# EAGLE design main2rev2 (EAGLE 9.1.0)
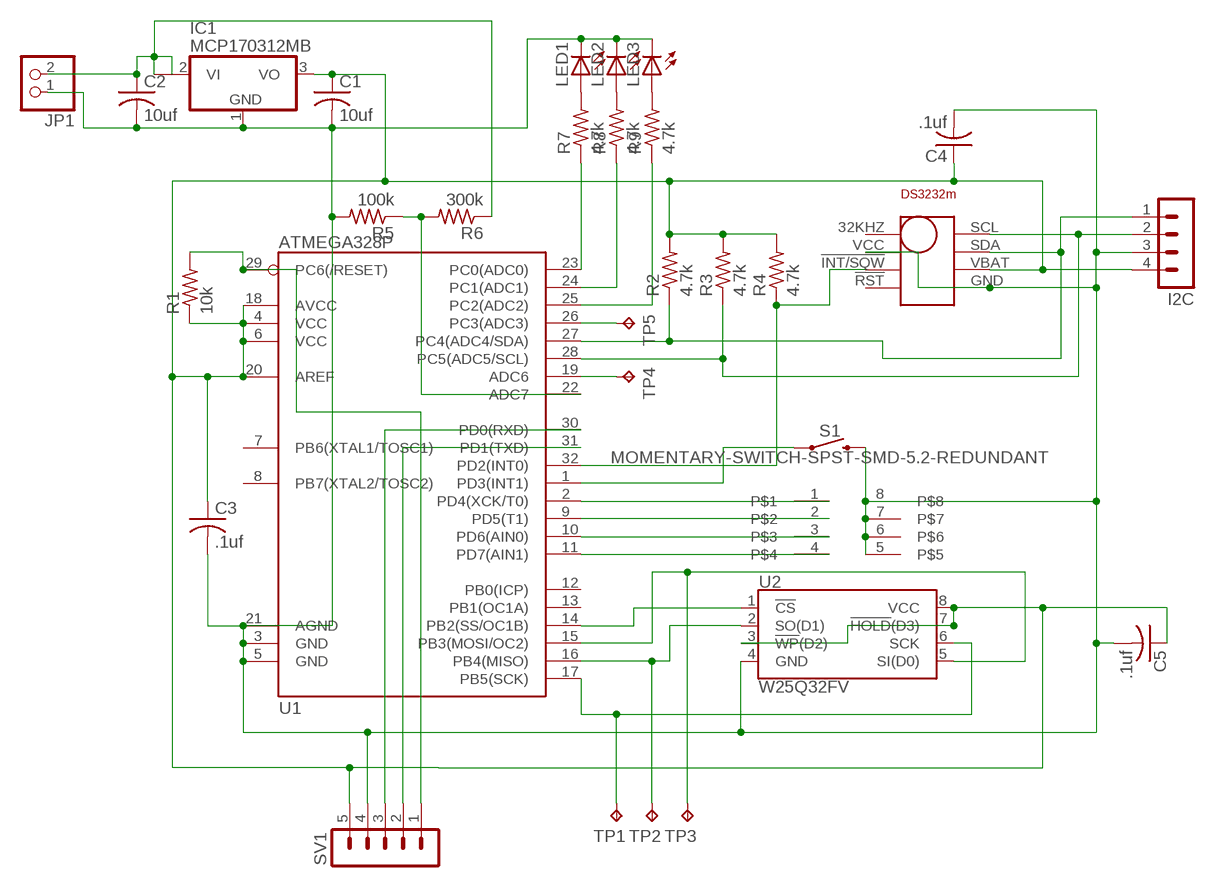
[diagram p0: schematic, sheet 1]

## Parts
C1  10uf  C-USC0805K  [C0805K]
C2  10uf  C-USC0805K  [C0805K]
C3  .1uf  C-USC0805K  [C0805K]
C4  .1uf  C-USC0805K  [C0805K]
C5  .1uf  C-USC0805K  [C0805K]
I2C  MA04-1  [MA04-1]
IC1  MCP170312MB  [SOT89]
JP1  PINHD-1X2  [1X02]
LED1  LEDSML0805  [SML0805]
LED2  LEDSML0805  [SML0805]
LED3  LEDSML0805  [SML0805]
R1  10k  R-US_R0805  [R0805]
R2  4.7k  R-US_R0805  [R0805]
R3  4.7k  R-US_R0805  [R0805]
R4  4.7k  R-US_R0805  [R0805]
R5  100k  R-US_R0805  [R0805]
R6  300k  R-US_R0805  [R0805]
R7  4.7k  R-US_R0805  [R0805]
R8  4.7k  R-US_R0805  [R0805]
R9  4.7k  R-US_R0805  [R0805]
S1  MOMENTARY-SWITCH-SPST-SMD-5.2-REDUNDANT  [TACTILE_SWITCH_SMD_5.2MM]
SV1  MA05-1  [MA05-1]
TP1  TPB1,27  [B1,27]
TP2  TPB1,27  [B1,27]
TP3  TPB1,27  [B1,27]
TP4  TPB1,27  [B1,27]
TP5  TPB1,27  [B1,27]
U1  ATMEGA328P  ATMEGA328_SMT  [TQFP32-08]
U2  W25Q32FV  W25Q32FVSS  [SOIC-8]
U$1  DS3232M  [SOIC8]
U$2  SO8-208  [SO08-208]

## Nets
N$1: S1.1 S1.2 U1.1(PD3(INT1))
N$2: TP1.TP U1.17(PB5(SCK)) U2.6(SCK)
N$3: R4.1 U1.32(PD2(INT0)) U$1.!INT/!!SQW
N$4: R1.2 SV1.1 U1.29(PC6(/RESET))
N$5: TP3.TP U1.15(PB3(MOSI/OC2)) U2.5(SI(D0))
N$6: TP2.TP U1.16(PB4(MISO)) U2.2(SO(D1))
N$7: U1.14(PB2(SS/OC1B)) U2.1(!CS!)
N$8: I2C.1 R2.1 U1.27(PC4(ADC4/SDA)) U$1.SDA
N$9: I2C.2 R3.1 U1.28(PC5(ADC5/SCL)) U$1.SCL
N$10: SV1.3 U1.30(PD0(RXD))
N$11: U1.11(PD7(AIN1)) U$2.4
N$12: U1.10(PD6(AIN0)) U$2.3
N$13: U1.9(PD5(T1)) U$2.2
N$14: U1.2(PD4(XCK/T0)) U$2.1
N$15: C1.2 C2.2 C3.2 C4.2 C5.2 I2C.3 IC1.1(GND) JP1.1 LED1.C LED2.C LED3.C R5.2 S1.3 S1.4 SV1.4 U1.3(GND) U1.5(GND) U1.21(AGND) U2.4(GND) U$1.GND U$1.VCC U$2.5 U$2.6 U$2.7 U$2.8
N$16: SV1.2 U1.31(PD1(TXD))
N$18: R5.1 R6.2 U1.22(ADC7)
N$19: LED1.A R7.2
N$20: LED2.A R8.2
N$21: LED3.A R9.2
N$22: R7.1 U1.23(PC0(ADC0))
N$23: R8.1 U1.24(PC1(ADC1))
N$24: R9.1 U1.25(PC2(ADC2))
N$25: C2.1 IC1.2(VI) IC1.2@1(VI1) JP1.2 R6.1
N$26: TP4.TP U1.19(ADC6)
N$27: C1.1 C3.1 C4.1 C5.1 I2C.4 IC1.3(VO) R1.1 R2.2 R3.2 R4.2 SV1.5 U1.4(VCC) U1.6(VCC) U1.18(AVCC) U1.20(AREF) U2.3(!WP!(D2)) U2.7(!HOLD!(D3)) U2.8(VCC) U$1.VBAT
N$28: TP5.TP U1.26(PC3(ADC3))
Unconnected: U1.7(PB6(XTAL1/TOSC1)) U1.8(PB7(XTAL2/TOSC2)) U1.12(PB0(ICP)) U1.13(PB1(OC1A)) U$1.32KHZ U$1.!RST

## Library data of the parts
C1-C5 = resistor:C-US: CAPACITOR, American symbol
I2C = con-lstb:MA04-1: PIN HEADER; OC_FARNELL: unknown; OC_NEWARK: unknown
IC1 = linear:MCP1703*: 250 mA, 16V, Low Quiescent Current LDO Regulator Source: http://ww1.microchip.com/downloads/en/DeviceDoc/22049b.pdf
JP1 = pinhead:PINHD-1X2: PIN HEADER
LED1-LED3 = led:LED: LED
R1-R9 = resistor:R-US_: RESISTOR, American symbol
S1 = SparkFun-Switches:MOMENTARY-SWITCH-SPST: Momentary Switch (Pushbutton) - SPST; PROD_ID: SWCH-08247; SF_SKU: COM-08720
SV1 = con-lstb:MA05-1: PIN HEADER; OC_FARNELL: unknown; OC_NEWARK: unknown
TP1-TP5 = testpad:TP: Test pad
U1 = SparkFun-DigitalIC:ATMEGA328_SMT: 32-Pin Atmega328 part Commonly used on Arduino compatible boards Available in QFP and QFN packages TQFP is IC-09069 QFN is non-stock; PROD_ID: IC-09069
U2 = SparkFun-IC-Memory:W25Q32FV: W25Q32FV 32Mb (4MB) Serial Flash Memory The W25Q32FV support the standard Serial Peripheral Interface (SPI), Dual/Quad I/O SPI as well as 2-clocks instruction cycle Quad Peripheral Interface (QPI). 104MHz, SPI, 8-SOIC-EIAJ Datasheet SparkFun Products SparkFun Blynk Board - ESP8266 (WRL-13794); PROD_ID: IC-13229
U$1 = DS3232M:DS3232M
U$2 = IC-packages_BIG-pack V1.0:SO8-208

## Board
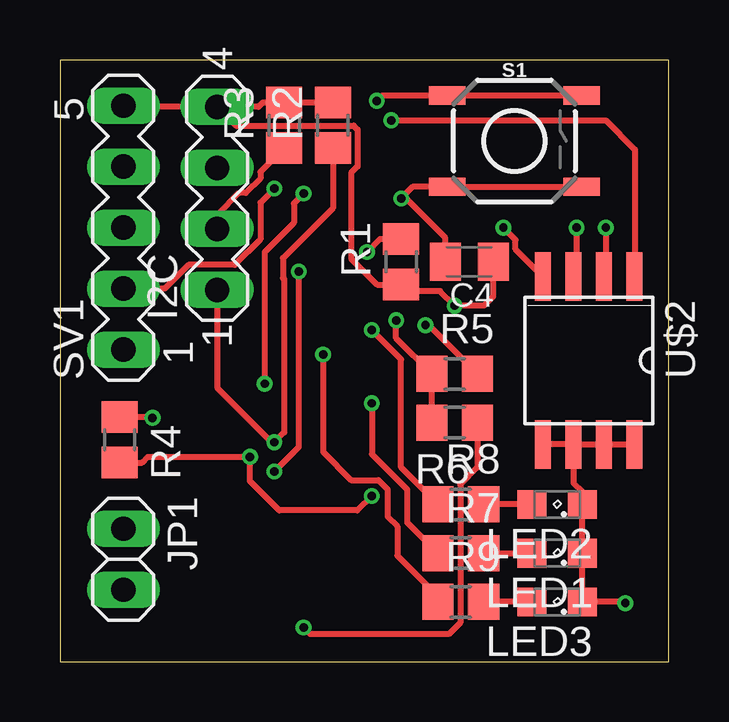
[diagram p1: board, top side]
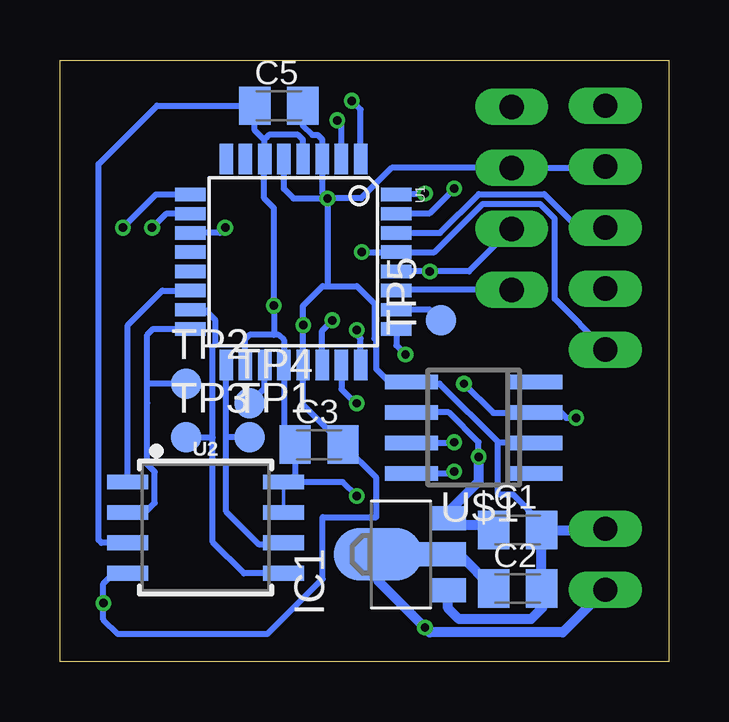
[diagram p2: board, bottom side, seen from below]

Size 25.38 x 25.07 mm. Coordinates in mm from the lower left corner, seen from the top.
Outline: 0,0 25.38,0 25.38,25.07 0,25.07 0,0
Copper layers (1*16): Top 0.035mm / dielectric 1.5mm / Bottom 0.035mm
Design rules "dirt_cheap_dirty_boards.v1.1": minimum track width 6mil, minimum drill 12mil, track to track 6mil, track to pad 6mil, pad to pad 6mil, via to via 6mil, smd to smd 0mil, copper to edge 10mil, drill to drill 10mil, minimum pad ring 10mil, minimum via ring 6mil, stop-mask expansion 2mil, vias tented up to drill 25mil, thermal gap 10mil

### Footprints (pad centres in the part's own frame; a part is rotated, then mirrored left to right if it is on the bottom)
C0805K = smd 1.3 x 1.6: 1 -1,0; 2 1,0
MA04-1 = drill 1.016 long: 1 -3.81,0; 2 -1.27,0; 3 1.27,0; 4 3.81,0
SOT89 = smd 1 x 1.5: 1 -1.499,-1.981; 3 1.499,-1.981 | smd 1 x 2: 2 0,-1.727 | smd 2.2 x 3.7: 2@1 0,0.94
1X02 = drill 1.016 long: 1 -1.27,0; 2 1.27,0
SML0805 = smd 1.2 x 1.2: A 1.05,0; C -1.05,0
R0805 = smd 1.3 x 1.5: 1 -0.95,0; 2 0.95,0
TACTILE_SWITCH_SMD_5.2MM = smd 1.524 x 0.762: 1 -2.794,1.905; 2 2.794,1.905; 3 -2.794,-1.905; 4 2.794,-1.905
MA05-1 = drill 1.016 long: 1 -5.08,0; 2 -2.54,0; 3 0,0; 4 2.54,0; 5 5.08,0
B1,27 = smd 1.27 x 1.27: TP 0,0
TQFP32-08 = smd 1.27 x 0.559: 1 -4.293,2.8; 2 -4.293,2; 3 -4.293,1.2; 4 -4.293,0.4; 5 -4.293,-0.4; 6 -4.293,-1.2; 7 -4.293,-2; 8 -4.293,-2.8; 17 4.293,-2.8; 18 4.293,-2; 19 4.293,-1.2; 20 4.293,-0.4; 21 4.293,0.4; 22 4.293,1.2; 23 4.293,2; 24 4.293,2.8 | smd 0.559 x 1.27: 9 -2.8,-4.293; 10 -2,-4.293; 11 -1.2,-4.293; 12 -0.4,-4.293; 13 0.4,-4.293; 14 1.2,-4.293; 15 2,-4.293; 16 2.8,-4.293; 25 2.8,4.293; 26 2,4.293; 27 1.2,4.293; 28 0.4,4.293; 29 -0.4,4.293; 30 -1.2,4.293; 31 -2,4.293; 32 -2.8,4.293
SOIC-8 = smd 0.61 x 1.702: 1 -1.905,-3.251; 2 -0.635,-3.251; 3 0.635,-3.251; 4 1.905,-3.251; 5 1.905,3.251; 6 0.635,3.251; 7 -0.635,3.251; 8 -1.905,3.251
SOIC8 = smd 0.6 x 2.2: 32KHZ -1.905,-2.6; !INT/!!SQW 0.635,-2.6; !RST 1.905,-2.6; GND 1.905,2.6; SCL -1.905,2.6; SDA -0.635,2.6; VBAT 0.635,2.6; VCC -0.635,-2.6
SO08-208 = smd 0.66 x 2.032: 1 -1.905,-3.498; 2 -0.635,-3.498; 3 0.635,-3.498; 4 1.905,-3.498; 5 1.905,3.498; 6 0.635,3.498; 7 -0.635,3.498; 8 -1.905,3.498

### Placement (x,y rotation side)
C1  6.3,5.49 0 bottom
C2  6.3,3.05 0 bottom
C3  14.58,9.04 0 bottom
C4  17.07,16.66 180 top
C5  16.26,23.16 0 bottom
I2C  6.55,19.3 90 top
IC1  11.18,4.47 90 bottom
JP1  2.64,4.27 270 top
LED1  20.73,4.52 180 top
LED2  20.73,6.55 180 top
LED3  20.73,2.49 180 top
R1  14.22,16.66 90 top
R2  11.38,22.35 90 top
R3  9.35,22.35 90 top
R4  2.49,9.25 270 top
R5  16.46,11.99 0 top
R6  16.46,9.96 180 top
R7  16.71,4.52 0 top
R8  16.71,6.55 0 top
R9  16.71,2.49 0 top
S1  18.95,21.69 0 top
SV1  2.64,18.08 90 top
TP1  17.48,9.35 0 bottom
TP2  20.12,11.58 0 bottom
TP3  20.12,9.35 0 bottom
TP4  17.48,10.77 0 bottom
TP5  9.5,14.22 90 bottom
U1  15.65,16.66 270 bottom
U2  19.3,5.59 270 bottom
U$1  8.13,9.75 90 bottom
U$2  22.05,12.55 180 top

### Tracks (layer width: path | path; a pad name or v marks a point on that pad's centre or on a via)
N$1  (via drill 0.35)
  Top 0.254: v13.21,23.37 13.44,23.6 S1.1 S1.2
  Bottom 0.254: U1.1 12.85,23.01 v13.21,23.37
N$2
  Bottom 0.254: U2.6 16.13,4.88 17.07,4.88 18.45,6.25 18.45,9.35 | 18.45,9.35 U1.17 | TP1.TP 18.45,9.35
N$3  (via drill 0.35)
  Top 0.254: v10.16,19.51 9.75,19.1 9.75,18.29 8.53,17.07 v8.53,11.58 | R4.1 3.83,10.2 v3.86,10.16
  Bottom 0.254: U1.32 11.31,19.51 v10.16,19.51 | v8.53,11.58 7.32,10.36 5.55,10.36 U$1.!INT/!!SQW 4.5,10.39 4.27,10.16 v3.86,10.16
N$4  (via drill 0.35)
  Top 0.254: v12.8,17.07 13.35,17.61 R1.2
  Bottom 0.254: v12.8,17.07 U1.29 9.76,17.06 7.75,19.07 5.36,19.07 4.75,18.46 4.75,15.11 SV1.1
N$5
  Bottom 0.254: U2.5 17.7,3.68 19,4.98 19,9.35 | 19,9.35 19,13.12 18.9,13.23 18.9,14.22 19.34,14.66 U1.15 | TP3.TP 19,9.35
N$6
  Bottom 0.254: U2.2 21.82,6.22 21.43,6.62 21.43,7.91 21.74,8.23 21.74,10.77 21.74,11.58 | 21.74,11.58 21.74,13.61 21.49,13.86 U1.16 | TP2.TP 21.74,11.58
N$7
  Bottom 0.254: U2.1 22.55,14.02 21.11,15.46 U1.14
N$8  (via drill 0.35)
  Top 0.254: I2C.1 6.55,11.41 8.82,9.14 v8.94,9.14 9.35,9.55 9.35,15.94 9.3,15.98 9.3,16.82 11.38,18.9 R2.1
  Bottom 0.254: I2C.1 11.32,15.49 U1.27 | U$1.SDA 8.91,9.12 v8.94,9.14
N$9  (via drill 0.35)
  Top 0.254: I2C.2 6.55,18.61 7.48,19.53 7.75,19.53 8.36,20.14 8.36,20.41 R3.1 | v9.96,16.26 9.96,8.94 v8.94,7.92
  Bottom 0.254: I2C.2 8.32,16.26 v9.95,16.26 v9.96,16.26 U1.28 | v8.94,7.92 9.02,7.85 U$1.SCL
N$10
  Bottom 0.254: SV1.3 2.86,17.86 3.57,17.86 5.19,19.48 7.92,19.48 9.53,17.86 U1.30
N$11  (via drill 0.35)
  Top 0.254: U$2.4 19,17.19 19,17.58 v18.49,18.09 | v18.49,18.09
  Bottom 0.254: v18.49,18.09 18.71,17.86 U1.11
N$12  (via drill 0.35)
  Top 0.254: v21.54,18.09 21.54,16.17 U$2.3
  Bottom 0.254: U1.10 20.96,18.66 v21.54,18.09
N$13  (via drill 0.35)
  Top 0.254: v22.76,18.09 22.76,16.12 U$2.2
  Bottom 0.254: U1.9 21.38,19.46 v22.76,18.09
N$14  (via drill 0.35)
  Top 0.254: v13.82,22.55 22.76,22.55 23.98,21.34 23.98,16.07 U$2.1
  Bottom 0.254: U1.2 13.65,22.38 v13.82,22.55
N$15  (via drill 0.35)
  Top 0.254: C4.2 16.07,17.66 14.43,19.3 v14.22,19.3 14.71,19.79 S1.3 S1.4 | R5.2 15.38,14.02 v15.24,14.02 | U$2.6 21.41,7.44 21.78,7.08 LED2.C LED1.C LED3.C 23.52,2.49 v23.57,2.44 | U$2.6 U$2.5 | U$2.6 U$2.7 U$2.8
  Bottom 0.254: U$1.VCC 7.09,9.12 | 7.09,9.12 7.11,9.09 7.11,6.97 6.5,6.97 5.3,5.77 C1.2 | U1.5 16.05,19.7 15.65,19.3 v14.22,19.3 | C5.2 15.26,22.33 14.87,21.95 14.63,21.95 14.45,21.76 U1.3 14.43,20.94 14.43,19.51 v14.22,19.3 | SV1.4 2.69,20.57 I2C.3 11.55,20.57 12.82,19.3 v14.22,19.3 | 14.43,3.45 | 7.09,9.12 9.55,11.58 9.96,11.58 10.03,11.66 U$1.GND 11.66,11.66 12.19,12.19 12.19,13.39 12.27,13.47 12.27,14.91 13.01,15.65 14.22,15.65 | 14.22,15.65 14.43,15.65 15.25,14.83 | 15.25,14.83 | 15.25,14.83 15.24,14.82 v15.24,14.02 v15.25,14.01 U1.21 15.24,10.7 C3.2 12.19,7.66 12.19,6.02 14.43,6.02 14.43,3.45 | 14.43,3.45 | 14.43,3.45 | 14.43,3.45 16.74,1.14 22.96,1.14 23.57,1.75 v23.57,2.44 23.57,3.25 23.14,3.68 U2.4 | v14.22,19.3 14.22,15.65
  Bottom 0.406: IC1.1 9.2,2.23 8.74,1.78 5.74,1.78 5.28,2.23 5.3,2.25 C2.2 C1.2 2.69,5.49 JP1.1
N$16  (via drill 0.35)
  Top 0.254: v8.94,19.71 8.36,19.13 8.36,17.6 7.29,16.54 5.36,16.54 4.37,15.54 SV1.2
  Bottom 0.254: U1.31 11.32,18.69 9.96,18.69 v8.94,19.71
N$18  (via drill 0.35)
  Top 0.254: v14.02,14.22 14.02,13.48 R5.1 R6.2
  Bottom 0.254: U1.22 14.45,13.8 v14.02,14.22
N$19
  Top 0.254: R7.2 LED1.A
N$20
  Top 0.254: LED2.A R8.2
N$21
  Top 0.254: LED3.A R9.2
N$22  (via drill 0.35)
  Top 0.254: v13.01,10.77 13.01,8.65 14.47,7.18 14.47,5.81 R7.1
  Bottom 0.254: v13.01,10.77 13.06,10.77 13.65,11.35 U1.23
N$23  (via drill 0.35)
  Top 0.254: R8.1 14.22,8.09 14.22,12.6 v13.01,13.82
  Bottom 0.254: U1.24 12.85,13.46 13.01,13.61 v13.01,13.82
N$24  (via drill 0.35)
  Top 0.254: v10.97,12.8 10.97,8.74 12.14,7.57 13.28,7.57 13.66,7.18 13.66,6.05 14.07,5.64 14.07,4.42 15.76,2.73 R9.1
  Bottom 0.254: U1.25 11.35,13.18 v10.97,12.8
N$25  (via drill 0.35)
  Top 0.254: R6.1 17.41,8.09 16.69,7.38 16.69,1.62 16.21,1.14 10.44,1.14 v10.16,1.42
  Bottom 0.254: IC1.2 10.16,4.47 IC1.2@1
  Bottom 0.406: JP1.2 4.42,1.22 9.96,1.22 v10.16,1.42 12.12,3.38 IC1.2@1 | IC1.2 8.72,4.47 C2.1
N$26
  Bottom 0.254: TP4.TP 16.85,11.4 U1.19
N$27  (via drill 0.35)
  Top 0.254: v13.01,6.91 12.39,6.3 9.14,6.3 7.92,7.52 v7.92,8.53 3.66,8.53 3.42,8.3 R4.2 | R2.2 R3.2 8.47,23.3 8.28,23.11 I2C.4 | C4.1 18.07,15.22 17.68,14.83 v16.46,14.83 15.85,15.44 14.7,15.44 14.43,15.71 R1.1 13.23,15.71 12.14,16.8 12.14,20.37 12.41,20.64 12.41,22.17 12.24,22.33 7.34,22.33 I2C.4 | I2C.4 2.69,23.11 SV1.5
  Bottom 0.152: U2.8 U2.7
  Bottom 0.254: 16.87,20.94 U1.6 | 16.46,13.61 16.26,13.61 16.05,13.4 U1.20 16.05,9.51 | 16.46,13.61 17.48,13.61 17.68,13.41 17.68,12.4 U1.18 | 16.46,13.61 v16.46,14.83 16.46,18.9 16.87,19.3 16.87,20.94 | v7.92,8.53 7.92,9.14 9.17,10.39 U$1.VBAT | U1.4 15.25,21.75 15.44,21.95 16.66,21.95 16.76,21.84 16.87,21.74 | 16.87,21.74 16.87,20.94 | 16.87,21.74 17.26,22.13 C5.1 21.34,23.16 23.77,20.73 23.77,5.08 23.65,4.95 U2.3 | U2.8 15.85,7.49 | 15.85,7.49 13.59,7.49 v13.01,6.91 | 16.05,9.51 C3.1 | C3.1 15.58,7.76 15.85,7.49 | 16.05,9.51 C3.1
  Bottom 0.406: v7.92,8.53 7.92,7.5 9.2,6.23 IC1.3 8.79,5.97 8.51,5.69 7.5,5.69 C1.1
N$28
  Bottom 0.254: TP5.TP 9.94,14.66 U1.26

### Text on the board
225bmp: XLII | Alnwlsn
